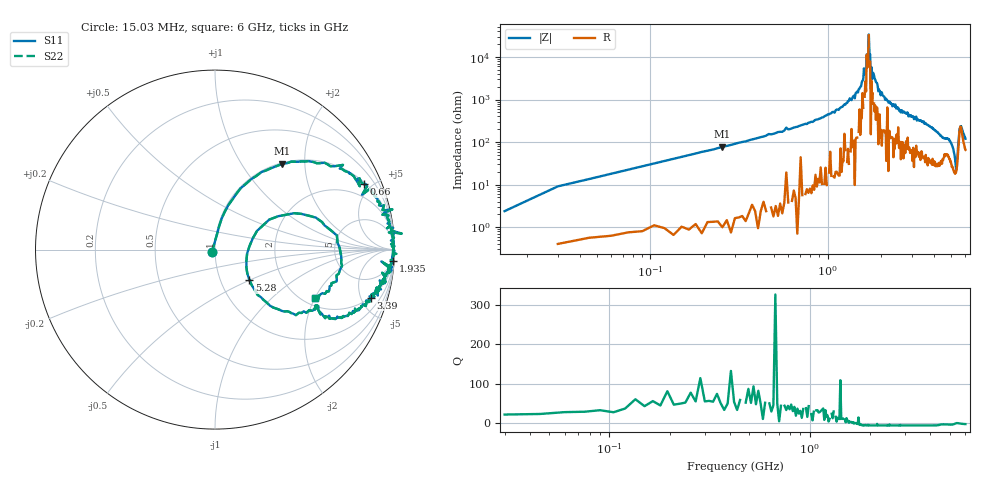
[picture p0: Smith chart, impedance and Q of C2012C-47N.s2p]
!	Network	Analyzer	HP8753E.07.74:	Oct	30	2002	Serial	No.	JP38451487
!	Hewlett-Packard
!	7	Sep	2009	10:56:05
!	Frequency	S11	S21	S12	S22
#	HZ	S	RI	R	50
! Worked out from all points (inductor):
!   400 points, 15.03 MHz to 6 GHz, reference 50 ohm
!   read as one part in series: L = 47.6 nH near 45.03 MHz
!   highest Q = 55.8 at 255 MHz (marker M1), where L = 48.3 nH
!   self-resonance near 1.65 GHz
!   S11 on the Smith chart (normalised r, x): 15.03 MHz: 0.97, -0.03; 660 MHz: 1.10, +4.50; 1.935 GHz: 3, -31; 3.39 GHz: 1.95, -6.06; 5.28 GHz: 1.37, -0.50; 6 GHz: 2.31, -2.01
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1.502992e7  -0.0174 -0.0154  1.02 0.0154  1.02 0.0154  -0.0174 -0.0154
3.002985e7  0.0122 0.0894  0.988 -0.0894  0.988 -0.0894  0.0122 0.0894
7.502962e7  0.0542 0.21  0.946 -0.21  0.946 -0.21  0.0542 0.21
2.550287e8  0.376 0.478  0.624 -0.478  0.624 -0.478  0.376 0.478
6.600267e8  0.83 0.365  0.17 -0.365  0.17 -0.365  0.83 0.365
1.020025e9  0.945 0.207  0.0546 -0.207  0.0546 -0.207  0.945 0.207
1.545022e9  0.989 0.0472  0.0107 -0.0472  0.0107 -0.0472  0.989 0.0472
1.695022e9  0.993 0.00668  0.00711 -0.00668  0.00711 -0.00668  0.993 0.00668
1.710021e9  0.997 0.000854  0.00281 -0.000854  0.00281 -0.000854  0.997 0.000854
1.740021e9  0.994 -0.00635  0.00574 0.00635  0.00574 0.00635  0.994 -0.00635
1.755021e9  0.995 0.0423  0.00458 -0.0423  0.00458 -0.0423  0.995 0.0423
1.770021e9  0.992 -0.0149  0.00839 0.0149  0.00839 0.0149  0.992 -0.0149
1.93502e9  0.992 -0.0632  0.00766 0.0632  0.00766 0.0632  0.992 -0.0632
2.01002e9  0.987 -0.0663  0.0132 0.0663  0.0132 0.0663  0.987 -0.0663
3.015015e9  0.925 -0.222  0.0746 0.222  0.0746 0.222  0.925 -0.222
3.390013e9  0.87 -0.267  0.13 0.267  0.13 0.267  0.87 -0.267
4.00501e9  0.761 -0.359  0.239 0.359  0.239 0.359  0.761 -0.359
5.010005e9  0.463 -0.356  0.537 0.356  0.537 0.356  0.463 -0.356
5.280004e9  0.192 -0.17  0.808 0.17  0.808 0.17  0.192 -0.17
5.460003e9  0.442 0.203  0.558 -0.203  0.558 -0.203  0.442 0.203
5.625002e9  0.702 -0.0281  0.298 0.0281  0.298 0.0281  0.702 -0.0281
6e9  0.558 -0.268  0.442 0.268  0.442 0.268  0.558 -0.268
